FUNCTION_BLOCK Example19_force // 1 flyway (actual physical) w/ 1 xbots - force mode ctrl,read payload,weigh xbot,read flyway temps
VAR_INPUT
	Execute : BOOL;
END_VAR
VAR_OUTPUT
	Done : BOOL;
END_VAR
VAR_IN_OUT
	PM_Controller : PMControllerType;	// the planar motor controller to use
END_VAR
VAR
	PMC_ForceModeCtrl1 : PMC_ForceModeCtrl;
	payload : REAL;
	PMC_WeighXbot1 : PMC_WeighXbotAsync;
	power : REAL;
	cpuTemp : REAL;
	PATemp : REAL;
	MTemp : REAL;
	PMC_GetFlywayStatus1 : PMC_GetFlywayStatus;
	Delay1 : Delay;
	PMC_ForceModeCtrl2 : PMC_ForceModeCtrl;
END_VAR

// 1 flyway (actual physical) w/ 1 xbots - force mode ctrl,read payload,weigh xbot,read flyway temps

//activate force mode control for xbot 1 in x axis 0 Newtons
PMC_ForceModeCtrl1(Execute := Execute,Mode := 0,Level := 2,Buffer := 0,XbotID := 1,ForceX := 0,ForceY := 0,ForceZ := 0,TorqueZ := 0,PM_Controller := PM_Controller);

//start the weighing process for xbot 1
PMC_WeighXbot1(Execute := PMC_ForceModeCtrl1.Done,XbotID := 1,Duration := 1.0,Weight => payload,PM_Controller := PM_Controller);

//lread power usage,CPU temp,amplifier temp, and motor temp of flyway 1
PMC_GetFlywayStatus1(Execute := PMC_WeighXbot1.Done,FlywayID := 1,Power => power,CPUTemp => cpuTemp,PATemp => PATemp,MTemp => MTemp,PM_Controller := PM_Controller);

//wait 10 seconds
Delay1(Execute := PMC_GetFlywayStatus1.Done,Cycles := 10000);

//exit force mode
PMC_ForceModeCtrl2(Execute := Delay1.Done,Mode := 0,Level := 0,XbotID := 1,ForceX := 0,ForceY := 0,ForceZ := 0,TorqueZ := 0,PM_Controller := PM_Controller);

Done := PMC_ForceModeCtrl2.Done;

END_FUNCTION_BLOCK
